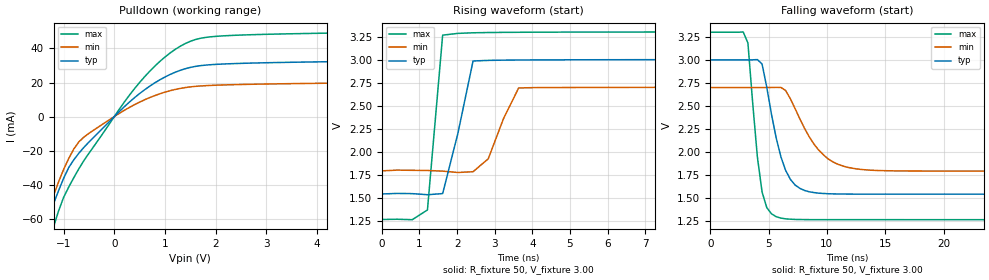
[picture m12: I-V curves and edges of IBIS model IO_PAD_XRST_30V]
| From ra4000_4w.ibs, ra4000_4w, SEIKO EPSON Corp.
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[Model]   IO_PAD_XRST_30V
Model_type Open_drain
Polarity Non-Inverting
Vref=3.30
Vmeas=1.50
Rref=5000
C_comp   2.5p   2.0p   3.0p
[Temperature Range] 25   125   -40
[Voltage Range]   3.00   2.70   3.30
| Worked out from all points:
|   slope of the pulldown table from 0 to 0.45 V, typ, clamps not added: 36.6 ohm
|   falling waveform, R_fixture 50, V_fixture 3.00: 20-80 % time 1.53ns typ, 2.57ns min, 918ps max; typ from 3 V to 1.54 V
|   rising waveform, R_fixture 50, V_fixture 3.00: 20-80 % time 488ps typ, 551ps min, 260ps max; typ from 1.54 V to 3 V
[Pulldown]
-3V       -244.2mA   -202.6mA   -296.9mA
-1.4V     -68.68mA   -63.41mA   -84.25mA
-1.3V     -59.72mA   -54.86mA   -74.25mA
-1.2V     -51.27mA   -46.4mA    -64.82mA
-900mV    -30mA      -24.64mA   -41.43mA
-600mV    -18.08mA   -12.07mA   -25.86mA
600mV     15.77mA    9.868mA    23.45mA
1.1V      24.7mA     15.17mA    37.31mA
1.5V      28.87mA    17.43mA    44.2mA
2.1V      30.79mA    18.51mA    47.31mA
5V        32.75mA    19.99mA    49.7mA
6V        34.91mA    21.45mA    52.66mA
[Falling Waveform]
R_fixture=50
V_fixture=3.00
V_fixture_min=2.70
V_fixture_max=3.30
0s        3V         2.7V       3.3V
2.828ns   3V         2.7V       3.303V
3.232ns   3V         2.7V       3.183V
4.04ns    3.003V     2.7V       1.949V
4.444ns   2.955V     2.7V       1.566V
5.657ns   2.151V     2.702V     1.298V
7.273ns   1.642V     2.471V     1.269V
9.293ns   1.554V     2.022V     1.266V
11.72ns   1.544V     1.835V     1.266V
40ns      1.543V     1.794V     1.266V
[Rising Waveform]
R_fixture=50
V_fixture=3.00
V_fixture_min=2.70
V_fixture_max=3.30
0s        1.543V     1.794V     1.266V
808.1ps   1.547V     1.799V     1.264V
1.212ns   1.535V     1.798V     1.37V
1.616ns   1.547V     1.791V     3.266V
2.02ns    2.198V     1.776V     3.285V
2.424ns   2.985V     1.784V     3.291V
2.828ns   2.992V     1.924V     3.294V
3.232ns   2.994V     2.358V     3.296V
3.636ns   2.996V     2.693V     3.297V
40ns      3V         2.7V       3.3V
[Ramp]
R_load=50
dV/dt_r   8.743E-1/2.876E-10   5.439E-1/4.875E-10   1.220E+0/1.754E-10
dV/dt_f   8.743E-1/1.516E-9   5.439E-1/2.563E-9   1.220E+0/8.753E-10
|[End   IO_PAD_XRST_30V
